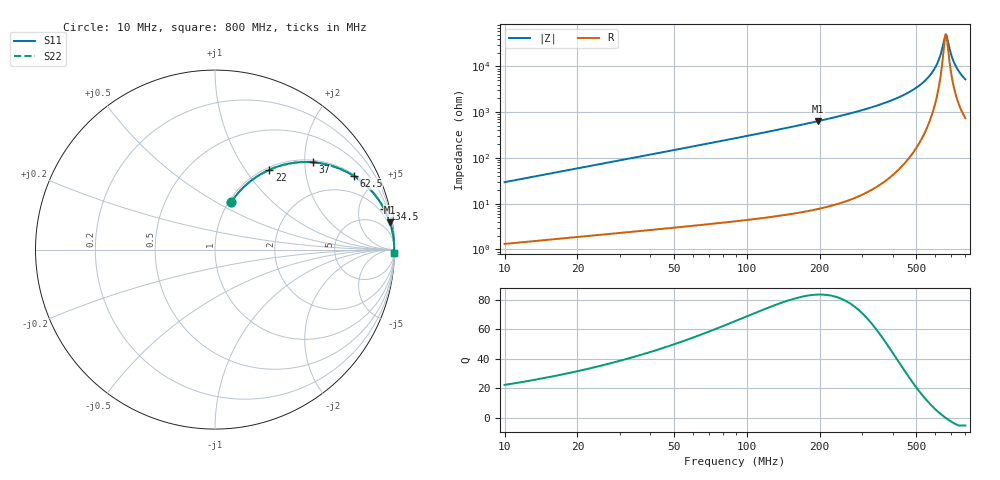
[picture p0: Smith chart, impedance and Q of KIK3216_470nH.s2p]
!version-2
!date-01.2022
!Series
# MHz S RI R 50
!Freq ReS11 ImS11 ReS21 ImS21 ReS12 ImS12 ReS22 ImS22
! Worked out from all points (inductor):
!   528 points, 10 MHz to 800 MHz, reference 50 ohm
!   read as one part in series: L = 470 nH near 13 MHz
!   highest Q = 83.5 at 197.5 MHz (marker M1), where L = 516 nH
!   self-resonance near 664 MHz
!   S11 on the Smith chart (normalised r, x): 10 MHz: 1.03, +0.59; 22 MHz: 1.04, +1.30; 37 MHz: 1.05, +2.19; 62.5 MHz: 1.07, +3.72; 134.5 MHz: 1.11, +8.28; 800 MHz: open
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10  0.0903 0.2652  0.9097 -0.2652  0.9097 -0.2652  0.0903 0.2652
22  0.3029 0.4447  0.6971 -0.4447  0.6971 -0.4447  0.3029 0.4447
37  0.5448 0.4865  0.4552 -0.4865  0.4552 -0.4865  0.5448 0.4865
49  0.6759 0.458  0.3241 -0.458  0.3241 -0.458  0.6759 0.458
62.5  0.7721 0.4105  0.2279 -0.4105  0.2279 -0.4105  0.7721 0.4105
91  0.8787 0.319  0.1213 -0.319  0.1213 -0.319  0.8787 0.319
134.5  0.9423 0.2268  0.0577 -0.2268  0.0577 -0.2268  0.9423 0.2268
142  0.9483 0.2152  0.0517 -0.2152  0.0517 -0.2152  0.9483 0.2152
197.5  0.9744 0.152  0.0256 -0.152  0.0256 -0.152  0.9744 0.152
274  0.9883 0.1012  0.0117 -0.1012  0.0117 -0.1012  0.9883 0.1012
406  0.9961 0.052  0.00394 -0.052  0.00394 -0.052  0.9961 0.052
481  0.9975 0.0334  0.00247 -0.0334  0.00247 -0.0334  0.9975 0.0334
538  0.998 0.0216  0.00197 -0.0216  0.00197 -0.0216  0.998 0.0216
578.5  0.9982 0.0141  0.00184 -0.0141  0.00184 -0.0141  0.9982 0.0141
608.5  0.9982 0.00898  0.00183 -0.00898  0.00183 -0.00898  0.9982 0.00898
634  0.9981 0.00481  0.00188 -0.00481  0.00188 -0.00481  0.9981 0.00481
659.5  0.998 0.000809  0.00197 -0.000809  0.00197 -0.000809  0.998 0.000809
668.5  0.998 -0.000565  0.00201 0.000565  0.00201 0.000565  0.998 -0.000565
694  0.9979 -0.00436  0.00215 0.00436  0.00215 0.00436  0.9979 -0.00436
718  0.9977 -0.00781  0.00231 0.00781  0.00231 0.00781  0.9977 -0.00781
754  0.9974 -0.0128  0.0026 0.0128  0.0026 0.0128  0.9974 -0.0128
800  0.997 -0.0188  0.00304 0.0188  0.00304 0.0188  0.997 -0.0188
